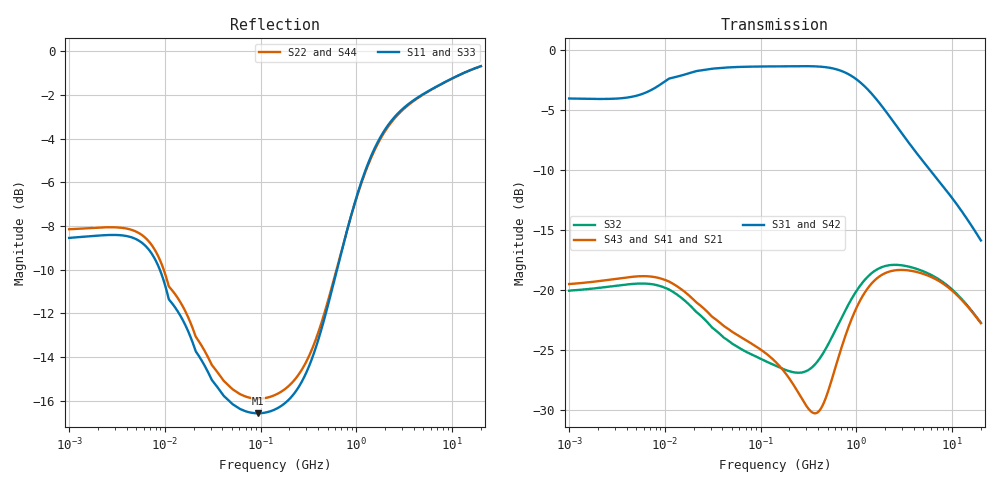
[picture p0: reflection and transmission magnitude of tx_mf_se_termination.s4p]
! Created Wed Jul 29 12:30:30 2015
# hz S db R 50
! 4 Port Network Data from SP1.SP block
! freq  dbS11  angS11  dbS12  angS12  dbS13  angS13  dbS14  angS14
!  dbS21  angS21  dbS22  angS22  dbS23  angS23  dbS24  angS24
!  dbS31  angS31  dbS32  angS32  dbS33  angS33  dbS34  angS34
!  dbS41  angS41  dbS42  angS42  dbS43  angS43  dbS44  angS44
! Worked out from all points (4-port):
!   861 points, 1 MHz to 20 GHz, reference 50 ohm
!   strongest paths, dB at 1 MHz, 11.89 MHz, 141.4 MHz, 1.682 GHz, 20 GHz:
!     S31: -4.0, -2.3, -1.4, -4.3, -15.9
!     S42: -4.3, -2.5, -1.5, -4.4, -15.9
!     S43: -19.5, -19.4, -25.9, -18.9, -22.7
!     S41: -19.5, -19.4, -25.9, -18.9, -22.7
!     S21: -19.5, -19.4, -25.9, -18.9, -22.7
!     S32: -20.0, -20.1, -26.3, -18.2, -22.7
!   lowest |S11| = -16.6 dB at 93.43 MHz (marker M1), VSWR 1.35, Z = 37.1 - j0.694 ohm
!   |S11| at or under -10 dB: 8.858 MHz to 628.3 MHz (619.5 MHz wide, 194 % of centre)
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1000000  -8.55 176.3  -20.03 -0.2  -4.05 2.2  -20.03 -0.2
         -19.48 0.2  -8.15 176.5  -19.48 0.2  -4.30 2.2
         -4.05 2.2  -20.03 -0.2  -8.55 176.3  -20.03 -0.2
         -19.48 0.2  -4.30 2.2  -19.48 0.2  -8.15 176.5
9445687  -10.33 157.9  -19.72 -18.5  -2.77 9.1  -19.72 -18.5
         -19.07 -16.1  -9.85 158.8  -19.07 -16.1  -2.98 9.4
         -2.77 9.1  -19.72 -18.5  -10.33 157.9  -19.72 -18.5
         -19.07 -16.1  -2.98 9.4  -19.07 -16.1  -9.85 158.8
9.342689e7  -16.58 -176.5  -25.60 -55.7  -1.39 -0.6  -25.60 -55.7
            -24.77 -43.7  -15.91 -177.2  -24.77 -43.7  -1.51 -0.5
            -1.39 -0.6  -25.60 -55.7  -16.58 -176.5  -25.60 -55.7
            -24.77 -43.7  -1.51 -0.5  -24.77 -43.7  -15.91 -177.2
3.720622e8  -13.65 -139.2  -26.15 -161.1  -1.38 -9.1  -26.15 -161.1
            -30.24 -148.6  -13.27 -142.4  -30.24 -148.6  -1.53 -9.1
            -1.38 -9.1  -26.15 -161.1  -13.65 -139.2  -26.15 -161.1
            -30.24 -148.6  -1.53 -9.1  -30.24 -148.6  -13.27 -142.4
1.887055e9  -3.75 -147.0  -18.05 44.6  -4.78 -37.8  -18.05 44.6
            -18.68 39.9  -3.83 -147.6  -18.68 39.9  -4.85 -37.1
            -4.78 -37.8  -18.05 44.6  -3.75 -147.0  -18.05 44.6
            -18.68 39.9  -4.85 -37.1  -18.68 39.9  -3.83 -147.6
6.396044e9  -1.69 -164.4  -18.83 -9.2  -10.35 -47.0  -18.83 -9.2
            -18.99 -9.7  -1.70 -164.3  -18.99 -9.7  -10.33 -46.8
            -10.35 -47.0  -18.83 -9.2  -1.69 -164.4  -18.83 -9.2
            -18.99 -9.7  -10.33 -46.8  -18.99 -9.7  -1.70 -164.3
2e10  -0.68 -171.5  -22.71 -40.0  -15.86 -58.0  -22.71 -40.0
      -22.74 -39.9  -0.68 -171.5  -22.74 -39.9  -15.85 -58.0
      -15.86 -58.0  -22.71 -40.0  -0.68 -171.5  -22.71 -40.0
      -22.74 -39.9  -15.85 -58.0  -22.74 -39.9  -0.68 -171.5
